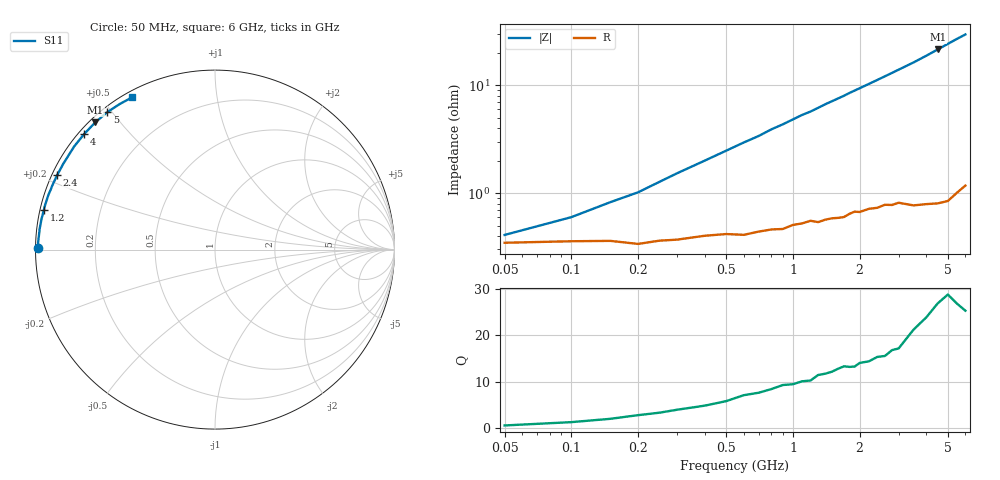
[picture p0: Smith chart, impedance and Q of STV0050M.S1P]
! SIEMENS Discrete & RF Semiconductors
! BA892
! Si PIN Diode in SCD-80
! IF = 50 mA
! S-Parameters:  September  1997
# GHz  S  MA  R  50
!  f  S11
! GHz  MAG  ANG
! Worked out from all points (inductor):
!   34 points, 50 MHz to 6 GHz, reference 50 ohm
!   read as one part to ground: L = 782 pH near 250 MHz
!   highest Q = 26.9 at 4.5 GHz (marker M1), where L = 763 pH
!   S11 on the Smith chart (normalised r, x): 50 MHz: 0.01, +0.00; 1.2 GHz: 0.01, +0.11; 2.4 GHz: 0.01, +0.22; 4 GHz: 0.02, +0.38; 5 GHz: 0.02, +0.49; 6 GHz: 0.02, +0.59
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0.05  0.9862 179.5
0.15  0.9857 178.3
0.2  0.9866 177.8
0.3  0.9853 176.6
0.5  0.9835 174.4
0.6  0.9838 173.3
0.7  0.9827 172.3
0.8  0.9819 171.1
0.9  0.9817 170.1
1.1  0.9795 167.9
1.2  0.9784 167.0
1.3  0.979 165.9
1.4  0.9779 164.8
1.6  0.9772 162.8
1.7  0.9769 161.8
1.8  0.9753 160.7
1.9  0.9742 159.7
2  0.9745 158.7
2.4  0.9726 154.7
2.6  0.971 152.7
2.8  0.9713 150.7
3  0.9702 148.7
3.5  0.9726 143.8
4  0.9727 138.6
4.5  0.9733 133.3
5  0.973 128.1
5.5  0.9692 123.1
6  0.9659 118.5
